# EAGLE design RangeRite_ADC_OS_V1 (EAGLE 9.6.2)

## Sheet 1 of 2: ADC Circuit
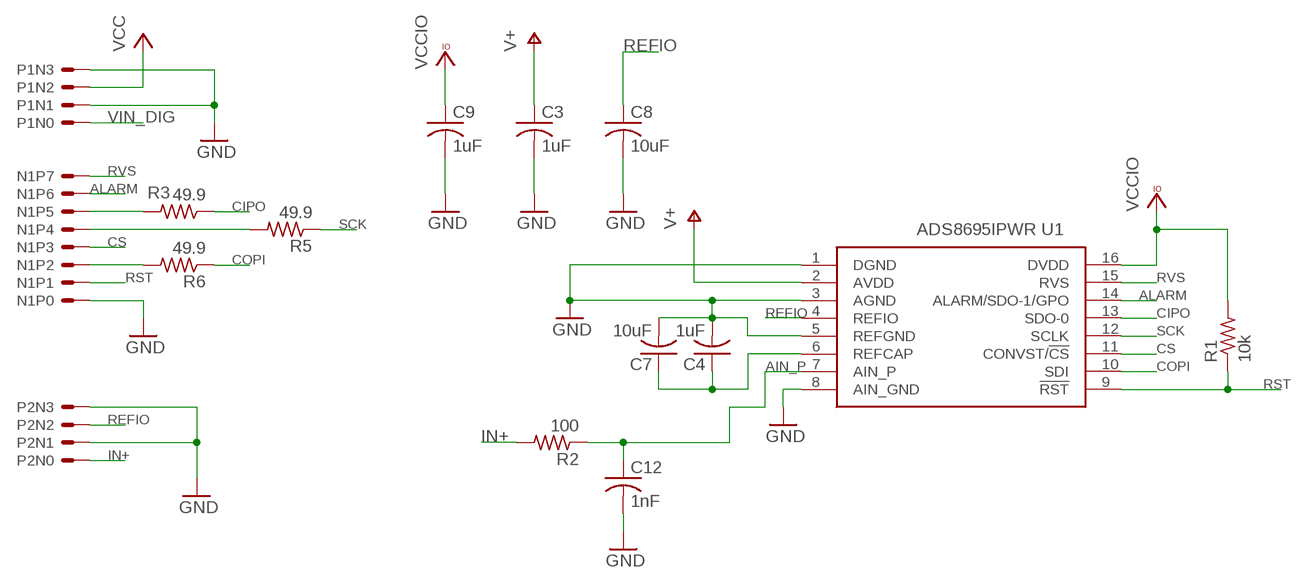
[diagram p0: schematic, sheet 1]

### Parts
C3  1uF  C-USC0603  [C0603]
C4  1uF  C-USC0603  [C0603]
C7  10uF  C-USC0603  [C0603]
C8  10uF  C-USC0603  [C0603]
C9  1uF  C-USC0603  [C0603]
C12  1nF  C-USC0603  [C0603]
N1  8PINHEADER  [8PINHEADER]
P1  4PINHEADER  [4PINHEADER]
P2  4PINHEADER  [4PINHEADER]
R1  10k  R-US_R0603  [R0603]
R2  100  R-US_R0603  [R0603]
R3  49.9  R-US_R0603  [R0603]
R5  49.9  R-US_R0603  [R0603]
R6  49.9  R-US_R0603  [R0603]
U1  ADS8695IPWR  [SOP65P640X120-16N]

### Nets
AIN_P: C12.1 R2.1 U1.7(AIN_P)
ALARM: N1.P6 U1.14(ALARM/SDO-1/GPO)
CIPO: R3.1 U1.13(SDO-0)
COPI: R6.1 U1.10(SDI)
CS: N1.P3 U1.11(CONVST/!CS)
GND: C3.2 C4.2 C7.2 C8.2 C9.2 C12.2 N1.P0 P1.N1 P1.N3 P2.N1 P2.N3 U1.1(DGND) U1.3(AGND) U1.5(REFGND) U1.8(AIN_GND) ; also sheet 2
IN+: P2.N0 R2.2
N$1: N1.P5 R3.2
N$2: C4.1 C7.1 U1.6(REFCAP)
N$3: N1.P4 R5.2
N$4: N1.P2 R6.2
REFIO: C8.1 P2.N2 U1.4(REFIO)
RST: N1.P1 R1.1 U1.9(!RST)
RVS: N1.P7 U1.15(RVS)
SCK: R5.1 U1.12(SCLK)
V+: C3.1 U1.2(AVDD) ; also sheet 2
VCC: P1.N2 ; also sheet 2
VCCIO: C9.1 R1.2 U1.16(DVDD) ; also sheet 2
VIN_DIG: P1.N0 ; also sheet 2

## Sheet 2 of 2: Power Circuits
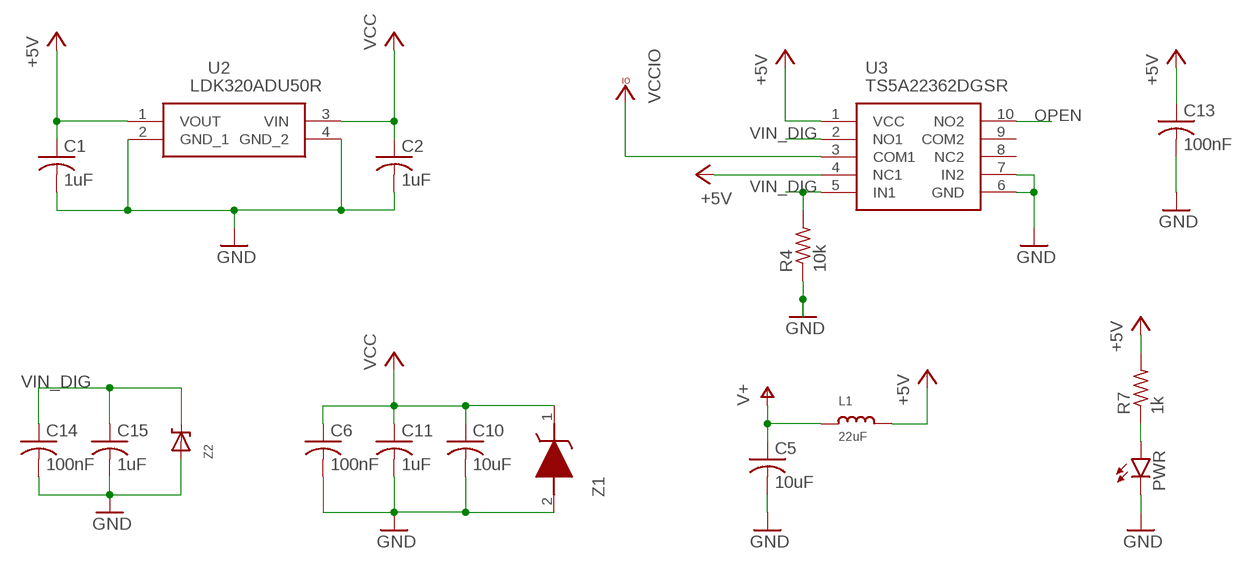
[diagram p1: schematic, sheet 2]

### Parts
C1  1uF  C-USC0603  [C0603]
C2  1uF  C-USC0603  [C0603]
C5  10uF  C-USC0603  [C0603]
C6  100nF  C-USC0603  [C0603]
C10  10uF  C-USC0805  [C0805]
C11  1uF  C-USC0603  [C0603]
C13  100nF  C-USC0603  [C0603]
C14  100nF  C-USC0603  [C0603]
C15  1uF  C-USC0603  [C0603]
L1  22uF  INDUCTOR0805  [0805]
PWR  LEDCHIP-LED0603  [CHIP-LED0603]
R4  10k  R-US_R0603  [R0603]
R7  1k  R-US_R0603  [R0603]
U2  LDK320ADU50R  [ST-SOT-89_1]
U3  TS5A22362DGSR  TS5A22364DGSR  [SOP50P490X110-10N]
Z1  MMSZ4706T1G  [SOD3716X135N]
Z2  DDZ5V6ASF  [DDZ5V6ASF]

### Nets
+5V: C1.1 C13.1 L1.2 R7.2 U2.1(VOUT) U3.1(VCC) U3.4(NC1)
GND: C1.2 C2.2 C5.2 C6.2 C10.2 C11.2 C13.2 C14.2 C15.2 PWR.C R4.1 U2.2(GND_1) U2.4(GND_2) U3.6(GND) U3.7(IN2) Z1.2(A) Z2.P$1(A) ; also sheet 1
N$5: PWR.A R7.1
OPEN: U3.10(NO2)
V+: C5.1 L1.1 ; also sheet 1
VCC: C2.1 C6.1 C10.1 C11.1 U2.3(VIN) Z1.1(K) ; also sheet 1
VCCIO: U3.3(COM1) ; also sheet 1
VIN_DIG: C14.1 C15.1 R4.2 U3.2(NO1) U3.5(IN1) Z2.P$2(C) ; also sheet 1
Unconnected: U3.8(NC2) U3.9(COM2)

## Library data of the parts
C1-C15 = rcl:C-US: CAPACITOR, American symbol; SPICEPREFIX: C
L1 = microbuilder:INDUCTOR: Inductors
N1 = ForceTronics:8PINHEADER: 8 pin header with 2.54mm spacing
P1 P2 = ForceTronics:4PINHEADER
PWR = led:LED: LED
R1-R7 = rcl:R-US_: RESISTOR, American symbol; SPICEPREFIX: R
U1 = SamacSys_Parts:ADS8695IPWR: 18-Bit, 500-kSPS, 1-Ch SAR ADC with programmable (+/-12/+/-10/+/-6/+/-5/+/-2.5V) input ranges on +5V supply Source: Datasheet; DESCRIPTION: 18-Bit, 500-kSPS, 1-Ch SAR ADC with programmable (+/-12/+/-10/+/-6/+/-5/+/-2.5V) input ranges on +5V supply; HEIGHT: 1.2mm; MANUFACTURER_NAME: Texas Instruments; MANUFACTURER_PART_NUMBER: ADS8695IPWR; MOUSER_PART_NUMBER: 595-ADS8695IPWR; MOUSER_PRICE-STOCK: https://www.mouser.co.uk/ProductDetail/Texas-Instruments/ADS8695IPWR?qs=34RfhUjJmKdJgoRRKR%252BX9g%3D%3D
U2 = SamacSys_Parts:LDK320ADU50R: LDO Voltage Regulators 200 mA low quiescent current and high PSRR voltage regulator Source: Datasheet; DESCRIPTION: LDO Voltage Regulators 200 mA low quiescent current and high PSRR voltage regulator; HEIGHT: mm; MANUFACTURER_NAME: STMicroelectronics; MANUFACTURER_PART_NUMBER: LDK320ADU50R; MOUSER_PART_NUMBER: 511-LDK320ADU50R; MOUSER_PRICE-STOCK: https://www.mouser.co.uk/ProductDetail/STMicroelectronics/LDK320ADU50R?qs=1mbolxNpo8cf%2F%2FtDZEZckA%3D%3D
U3 = SamacSys_Parts:TS5A22364DGSR: Analog Switch ICs 0.65-Ohm Dual SPDT Analog Switch Source: Datasheet; DESCRIPTION: Analog Switch ICs 0.65-Ohm Dual SPDT Analog Switch; HEIGHT: 1.1mm; MANUFACTURER_NAME: Texas Instruments; MANUFACTURER_PART_NUMBER: TS5A22364DGSR; MOUSER_PART_NUMBER: 595-TS5A22364DGSR; MOUSER_PRICE-STOCK: https://www.mouser.co.uk/ProductDetail/Texas-Instruments/TS5A22364DGSR?qs=9F2IyUQaA%2FhbjQmUI4VB%2FQ%3D%3D
Z1 = SamacSys_Parts:MMSZ4706T1G: 500 mW Rating on FR-4 or FR-5 Board; Wide Zener Reverse Voltage Range - 1.8 V to 43 V; Package Designed for Optimal Automated Board Assembly; Small Package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; DESCRIPTION: 500 mW Rating on FR-4 or FR-5 Board; Wide Zener Reverse Voltage Range - 1.8 V to 43 V; Package Designed for Optimal Automated Board Assembly; Small Package Size for High Density Applications; ESD Rating of Class 3 (exceeding 16 kV) per the Human Body Model Mechanical Characteristics:; CASE: Void-free, transfer-molded, thermosetting plastic case; FINISH: Corrosion resistant finish, easily solderable; MAXIMUM CASE TEMPERATURE FOR SOLDERING PURPOSES: 260?C for 10 Seconds; POLARITY: Cathode indicated by polarit; HEIGHT: 1.35mm; MANUFACTURER_NAME: onsemi; MANUFACTURER_PART_NUMBER: MMSZ4706T1G; MOUSER_PART_NUMBER: 863-MMSZ4706T1G; MOUSER_PRICE-STOCK: https://www.mouser.co.uk/ProductDetail/ON-Semiconductor/MMSZ4706T1G?qs=P4IOph%252Bbot%252BLTfzGd%2F4B3g%3D%3D
Z2 = ForceTronics-ForceTronics:DDZ5V6ASF: DDZ5V6ASF 5.42 Zener Diode

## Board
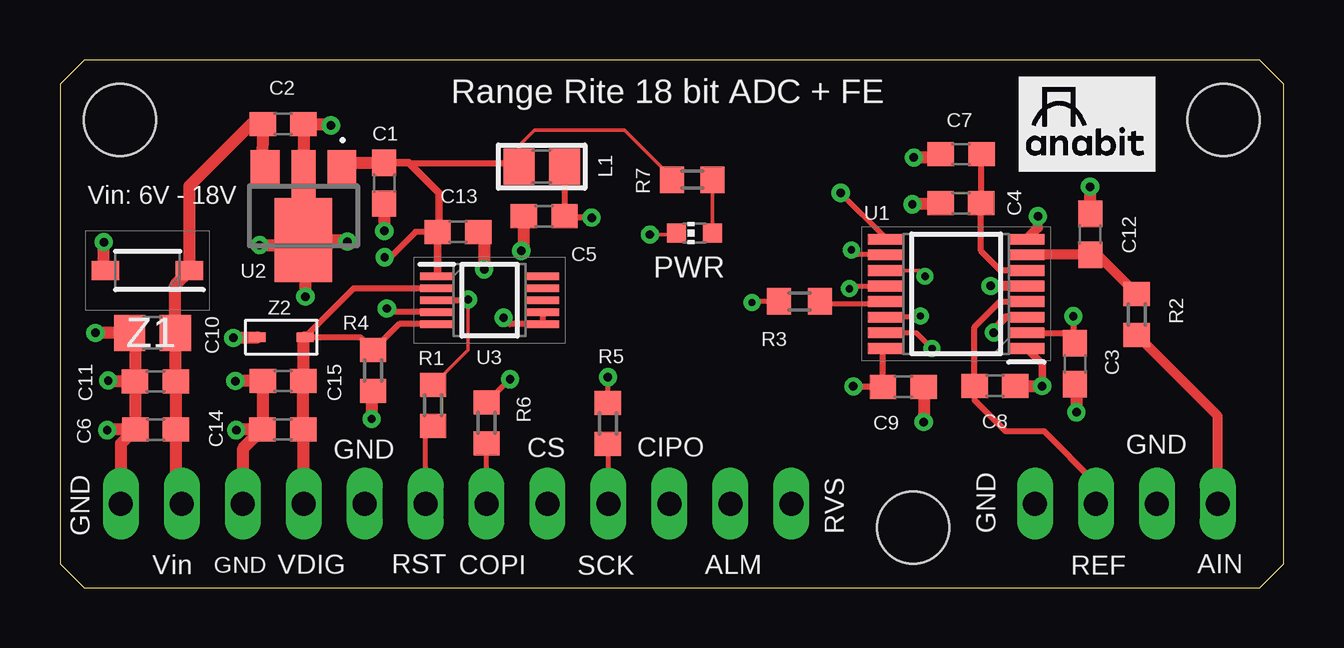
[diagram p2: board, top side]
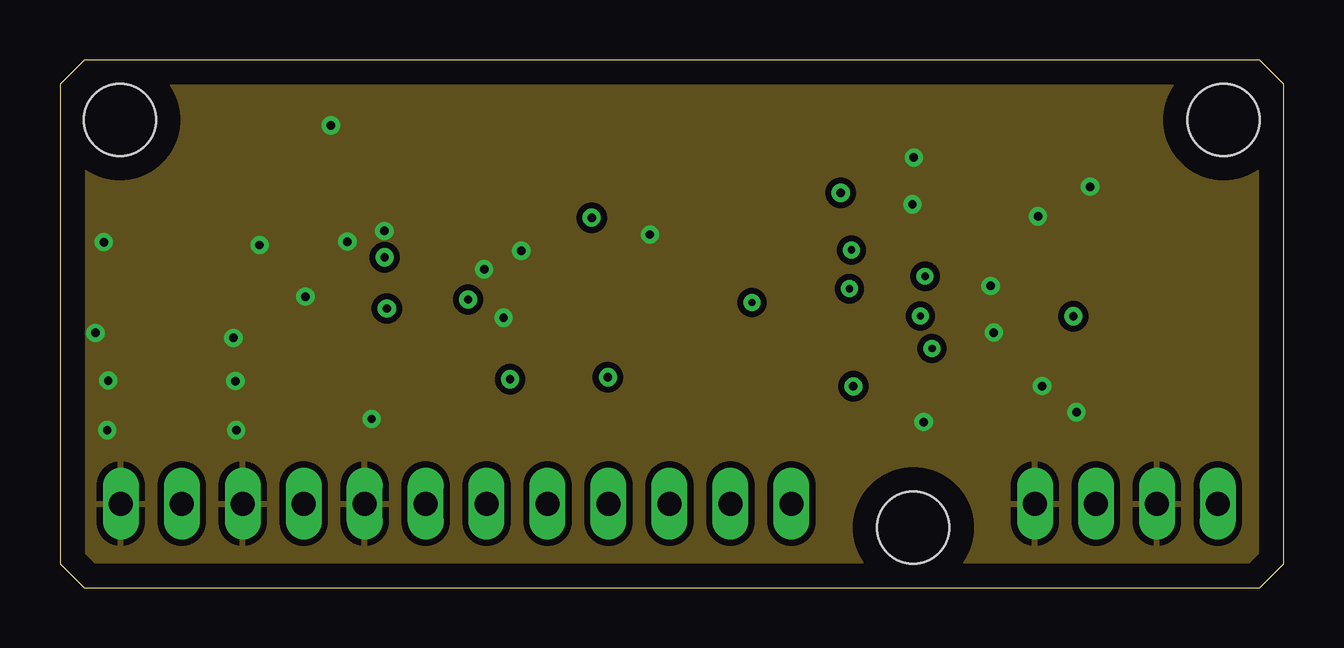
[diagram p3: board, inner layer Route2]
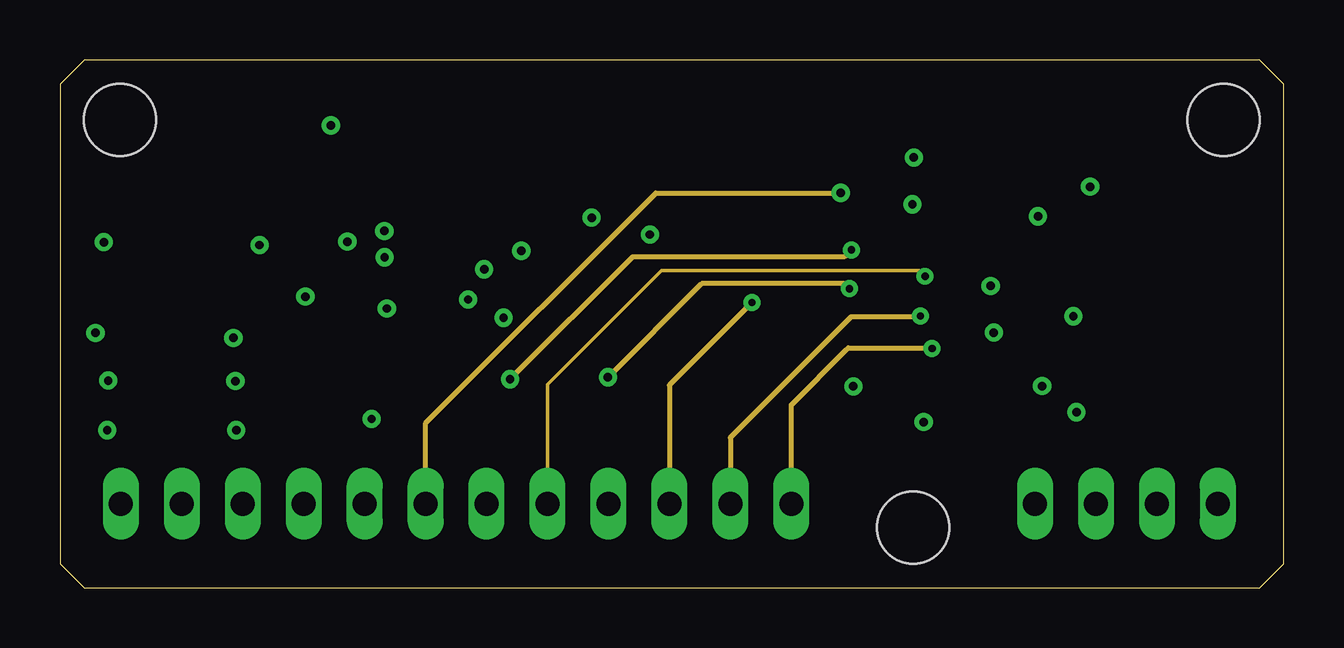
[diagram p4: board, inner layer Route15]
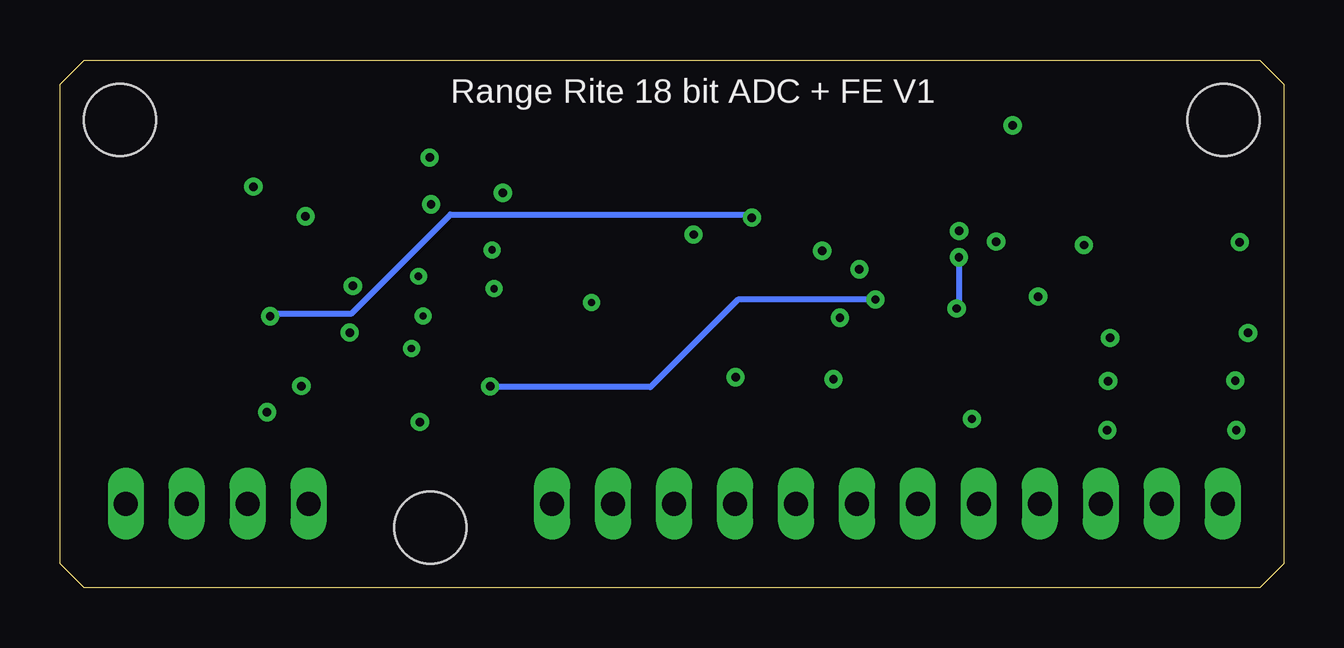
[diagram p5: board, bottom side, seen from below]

Size 51 x 22 mm. Coordinates in mm from the lower left corner, seen from the top.
Outline: 0,21 0,1 1,0 50,0 51,1 51,21 50,22 1,22 0,21
Copper layers (1+2*15+16): Top 0.035mm / dielectric 0.5mm / Route2 0.035mm / dielectric 0.5mm / Route15 0.035mm / dielectric 0.5mm / Bottom 0.035mm
Design rules "default *": minimum track width 6mil, minimum drill 0.3mm, track to track 6mil, track to pad 6mil, pad to pad 6mil, via to via 6mil, smd to smd 6mil, copper to edge 40mil, drill to drill 6mil, minimum pad ring 10mil, minimum via ring 8mil, stop-mask expansion 4mil, vias tented up to drill 0mil, thermal gap 10mil
Holes 3 mm at 35.57,2.5 2.5,19.5 48.5,19.5

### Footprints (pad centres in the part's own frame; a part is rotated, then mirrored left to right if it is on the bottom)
C0603 = smd 1.1 x 1: 1 -0.85,0; 2 0.85,0
C0805 = smd 1.3 x 1.5: 1 -0.95,0; 2 0.95,0
0805 = smd 1.3 x 1.5: 1 -0.95,0; 2 0.95,0
8PINHEADER = drill 1 long: P0 1.27,-3.81; P1 3.81,-3.81; P2 6.35,-3.81; P3 8.89,-3.81; P4 11.43,-3.81; P5 13.97,-3.81; P6 16.51,-3.81; P7 19.05,-3.81
4PINHEADER = drill 1 long: N0 -3.81,0; N1 -1.27,0; N2 1.27,0; N3 3.81,0
CHIP-LED0603 = smd 0.8 x 0.8: A 0,-0.75; C 0,0.75
R0603 = smd 1 x 1.1: 1 -0.85,0; 2 0.85,0
SOP65P640X120-16N = smd 1.475 x 0.45: 1 -2.938,2.275; 2 -2.938,1.625; 3 -2.938,0.975; 4 -2.938,0.325; 5 -2.938,-0.325; 6 -2.938,-0.975; 7 -2.938,-1.625; 8 -2.938,-2.275; 9 2.938,-2.275; 10 2.938,-1.625; 11 2.938,-0.975; 12 2.938,-0.325; 13 2.938,0.325; 14 2.938,0.975; 15 2.938,1.625; 16 2.938,2.275
ST-SOT-89_1 = smd 1.2 x 1.5: 1 -1.6,-2; 3 1.6,-2 | smd 1 x 2: 2 0,-1.75 | smd 2.4 x 3.5: 4 0,1
SOP50P490X110-10N = smd 1.4 x 0.3: 1 -2.2,1; 2 -2.2,0.5; 3 -2.2,0; 4 -2.2,-0.5; 5 -2.2,-1; 6 2.2,-1; 7 2.2,-0.5; 8 2.2,0; 9 2.2,0.5; 10 2.2,1
SOD3716X135N = smd 1.15 x 0.8: 1 -1.75,0; 2 1.75,0
DDZ5V6ASF = smd 0.71 x 0.41: P$1 0,0; P$2 1.99,0

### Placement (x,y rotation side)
C1  13.51,16.86 270 top
C2  9.3,19.32 0 top
C3  42.3,9.33 270 top
C4  37.55,16.03 180 top
C5  20.18,15.48 180 top
C6  3.99,6.59 180 top
C7  37.56,18.08 180 top
C8  38.97,8.41 0 top
C9  35.15,8.37 0 top
C10  3.86,10.62 180 top
C11  3.98,8.6 180 top
C12  42.95,14.73 90 top
C13  16.59,14.83 0 top
C14  9.29,6.6 180 top
C15  9.3,8.62 180 top
L1  20.08,17.55 180 top
N1  11.43,7.31 0 top
P1  6.35,3.5 180 top
P2  44.45,3.5 180 top
PWR  26.45,14.78 90 top
R1  15.55,7.6 90 top
R2  44.88,11.38 270 top
R3  30.82,11.93 180 top
R4  13.05,9.05 90 top
R5  22.84,6.84 270 top
R6  17.78,6.87 270 top
R7  26.35,17 180 top
U1  37.35,12.25 180 top
U2  10.15,15.5 180 top
U3  17.91,11.98 0 top
Z1  3.65,13.22 180 top
Z2  8.22,10.44 0 top

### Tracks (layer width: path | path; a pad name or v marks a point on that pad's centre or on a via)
+5V  (via drill 0.35)
  Top 0.152: L1.2 19.13,18.43 19.78,19.08 23.52,19.08 25.5,17.09 R7.2
  Top 0.254: C13.1 14.82,14.83 13.76,13.77 v13.53,13.77 | v13.62,11.63 13.78,11.48 15.44,11.48 U3.4 | 14.55,17.7 18.98,17.7 L1.2
  Top 0.305: C1.1 14.54,17.71 14.55,17.7 15.8,16.45 15.8,14.89 C13.1 15.74,13.01 U3.1
  Top 0.508: U2.1 11.96,17.71 C1.1
  Bottom 0.254: v13.53,13.77 13.53,11.69 13.59,11.63 v13.62,11.63
AIN_P
  Top 0.305: 40.3,13.89 U1.7
  Top 0.406: R2.1 43.23,13.88 C12.1 U1.7
ALARM  (via drill 0.3)
  Top 0.2: v35.86,11.32 35.81,11.28 U1.14
  Route15 0.2: 32.93,11.25 32.98,11.3 35.84,11.3 v35.86,11.32
  Route15 0.203: 32.93,11.25 27.94,6.26 N1.P6
CIPO
  Top 0.203: U1.13 34.3,11.81 31.79,11.81 R3.1
COPI  (via drill 0.3, 0.35)
  Top 0.203: R6.1 18.74,8.68 18.74,8.69 v18.76,8.69 | v32.99,14.08 33.19,13.88 U1.10
  Route15 0.203: v18.76,8.69 23.86,13.79 32.7,13.79 v32.99,14.08
CS  (via drill 0.3)
  Top 0.152: v36.06,12.98 35.81,13.22 U1.11
  Route15 0.152: N1.P3 20.32,8.47 25.07,13.22 35.82,13.22 v36.06,12.98
GND  (via drill 0.35)
  Top 0.152: PWR.C 25.64,14.72 v24.59,14.72
  Top 0.254: v40.93,8.41 v40.94,8.4 | v18.49,11.25 18.76,10.98 U3.6 U3.7
  Top 0.305: U1.3 39.44,11.28 38.92,10.76 v38.92,10.63 | U1.1 40.94,9.32 v40.94,8.4
  Top 0.406: U1.8 40.77,15 v40.77,15.48 | U1.5 v38.8,12.57 v38.79,12.58
  Top 0.508: Z1.2 1.83,13.29 v1.83,14.4 | C8.2 v40.93,8.41 | C3.2 42.37,8.41 v42.37,7.31 | C9.2 v36,6.9 | C12.2 42.94,15.57 v42.94,16.71 | C4.2 36.65,15.98 v35.53,15.98 | C7.2 36.56,17.93 v35.59,17.93 | v11.29,19.27 11.24,19.32 C2.2 U2.2 | v8.32,14.28 9.93,14.28 | 9.93,14.28 U2.4 11.9,14.5 v11.98,14.42 | v10.23,12.13 10.23,13.98 9.93,14.28 | C1.2 v13.52,14.87 | C13.2 17.68,14.59 v17.68,13.27 | C5.2 19.33,14.14 v19.23,14.04 | Z2.P$1 8.19,10.41 v7.23,10.41 | R4.1 12.99,8.14 v12.99,7.03 | v7.31,8.61 v7.32,8.62 C15.2 C14.2 | C14.2 7.39,6.6 v7.35,6.56 | C11.2 2.04,8.6 v2.01,8.63 | C6.2 2,6.59 v1.97,6.56 | v1.48,10.62 C10.2 3.13,10.4 C11.2 | C11.2 C6.2 | C6.2 2.54,5.99 P1.N3 | C14.2 7.62,5.78 P1.N1
  pour Route2 (isolate 0.254): -1,24 -1,-2 53,-2 53,24
IN+
  Top 0.406: P2.N0 48.26,7.15 R2.2
N$1  (via drill 0.3)
  Top 0.203: R3.2 29.1,11.93 29.05,11.88 v28.84,11.88
  Route15 0.203: v28.84,11.88 25.4,8.44 N1.P5
N$2
  Top 0.254: U1.6 39.2,13.22 38.39,14.04 C4.1 C7.1
N$3
  Top 0.203: N1.P4 22.86,5.97 R5.2
N$4
  Top 0.203: N1.P2 R6.2
N$5
  Top 0.152: R7.1 PWR.A
REFIO
  Top 0.254: U1.4 39.17,11.93 38.12,10.87 C8.1 38.12,7.82 39.41,6.53 41,6.53 43.18,4.35 P2.N2
RST  (via drill 0.35)
  Top 0.2: N1.P1 15.24,6.44 R1.1 | U1.9 34.41,14.59 v32.54,16.46
  Route15 0.2: N1.P1 15.24,6.86 24.84,16.46 v32.54,16.46
RVS  (via drill 0.3)
  Top 0.2: v36.35,9.97 35.7,10.62 U1.15
  Route15 0.2: 32.78,9.93 32.86,10 36.32,10 v36.35,9.97
  Route15 0.203: N1.P7 30.48,7.62 32.78,9.93
SCK  (via drill 0.3, 0.35)
  Top 0.203: R5.1 22.84,8.62 22.83,8.63 v22.83,8.76 v22.84,8.77 | v32.91,12.46 33.02,12.57 U1.12
  Route15 0.203: v22.84,8.77 26.75,12.68 32.7,12.68 v32.91,12.46
V+  (via drill 0.35)
  Top 0.254: U1.2 41.85,10.62 C3.1 42.24,10.24 v42.24,11.31 | L1.1 C5.1 21.08,15.43 v22.15,15.43 v22.16,15.42
  Bottom 0.254: v22.16,15.42 22.29,15.55 34.73,15.55 38.87,11.41 42.24,11.41 v42.24,11.31
VCC
  Top 0.508: P1.N2 4.84,3.74 C6.1 C11.1 4.83,10.6 C10.1 4.81,12.63 Z1.1 5.4,16.76 7.96,19.32 C2.1 8.45,19.24 8.48,19.21 8.41,17.6 U2.3
VCCIO  (via drill 0.35)
  Top 0.152: v17.01,12.01 17.01,9.91 R1.2
  Top 0.254: U1.16 34.3,9.86 C9.1 34.28,8.39 v33.07,8.39 | U3.3 16.98,11.98 v17.01,12.01
  Bottom 0.254: v17.01,12.01 22.74,12.01 26.39,8.36 33.07,8.36 v33.07,8.39
VIN_DIG
  Top 0.254: U3.5 14.13,10.98 R4.2 12.51,10.44 Z2.P$2 12.25,12.48 U3.2
  Top 0.508: P1.N0 10.16,6.58 C14.1 C15.1 10.15,10.38 Z2.P$2

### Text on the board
tNames: Range Rite 18 bit ADC + FE | Vin: 6V - 18V | GND | CS | CIPO | GND | RVS | GND | GND | Vin | GND | VDIG | RST | COPI | SCK | ALM | REF | AIN
bNames: Range Rite 18 bit ADC + FE V1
